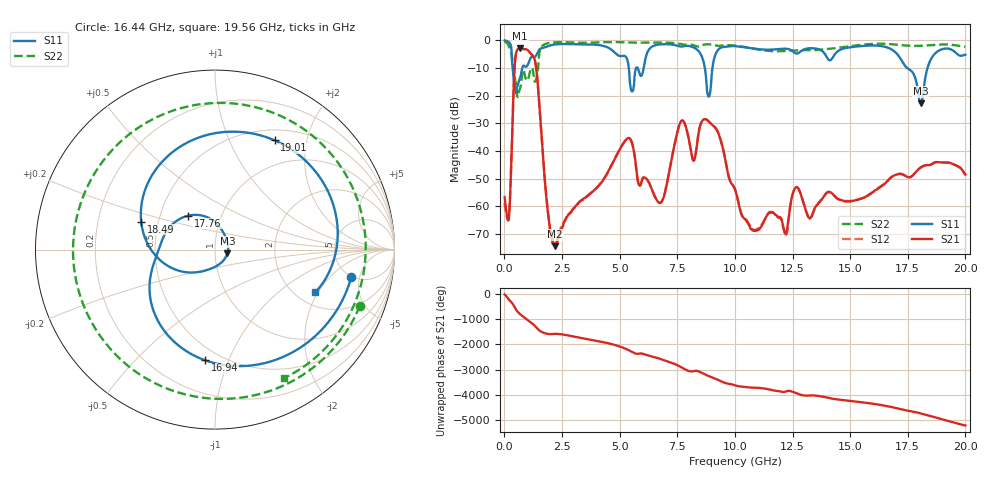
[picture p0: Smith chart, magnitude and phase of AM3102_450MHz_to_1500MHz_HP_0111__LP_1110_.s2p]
!Agilent Technologies,E8364B,MY43040894,A.07.50.67
!Agilent E8364B: A.07.50.67
!Date: Thursday, January 11, 2018 05:54:55
!Correction: S11(Full 2 Port(1,2))
!S21(Full 2 Port(1,2))
!S12(Full 2 Port(1,2))
!S22(Full 2 Port(1,2))
!S2P File: Measurements: S11, S21, S12, S22:
# Hz S  dB  R 50
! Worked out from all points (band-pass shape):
!   1601 points, 10 MHz to 20 GHz, reference 50 ohm
!   highest |S21| = -2.97 dB at 684.7 MHz (marker M1); lowest = -74.4 dB at 2.196 GHz (marker M2)
!   |S21| within 3 dB of the highest: 483.1 MHz to 1.265 GHz (781.5 MHz wide, 89.4 % of centre)
!   lowest |S11| = -22.9 dB at 18.06 GHz (marker M3), VSWR 1.16, Z = 57.3 - j2.44 ohm
!   |S11| at or under -10 dB: 358.2 MHz to 777.4 MHz (419.2 MHz wide, 73.8 % of centre); 8.697 GHz to 9.025 GHz (328.6 MHz wide, 3.71 % of centre); 17.47 GHz to 18.36 GHz (889.4 MHz wide, 4.97 % of centre)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
!   |S22| runs from -20.5 to -0.5 dB; largest |S21 - S12| = 0.0015
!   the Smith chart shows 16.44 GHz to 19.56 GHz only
!   S11 on the Smith chart (normalised r, x): 16.44 GHz: 4.90, -3.77; 16.94 GHz: 0.41, -0.83; 17.76 GHz: 0.70, +0.28; 18.49 GHz: 0.40, +0.16; 19.01 GHz: 0.64, +1.49; 19.56 GHz: 2.50, -1.89
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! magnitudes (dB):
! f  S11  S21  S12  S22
! 10 MHz  -0.1  -56.7  -58.9  -0.5
! 197.4 MHz  -0.7  -64.1  -63.4  -2.3
! 472.3 MHz  -17.8  -6.8  -6.8  -14.3
! 684.7 MHz  -13.5  -3.0  -3.0  -17.4
! 1.347 GHz  -5.8  -8.2  -8.2  -14.8
! 2.196 GHz  -1.5  -74.4  -73.7  -0.7
! 3.346 GHz  -1.5  -57.8  -57.9  -0.9
! 5.382 GHz  -9.0  -35.3  -35.3  -0.8
! 6.682 GHz  -1.6  -58.5  -58.5  -0.8
! 7.706 GHz  -2.3  -29.0  -29.0  -1.4
! 8.868 GHz  -20.3  -29.4  -29.4  -1.5
! 10.01 GHz  -2.1  -53.9  -53.9  -1.9
! 13.34 GHz  -2.9  -63.4  -63.5  -3.6
! 16.44 GHz  -2.2  -52.3  -52.2  -1.3
! 16.68 GHz  -2.8  -50.4  -50.3  -1.3
! 16.94 GHz  -4.2  -48.8  -48.8  -1.5
! 17.76 GHz  -12.4  -48.5  -48.5  -2.0
! 18.06 GHz  -22.9  -45.9  -46.0  -2.0
! 18.49 GHz  -7.1  -45.0  -45.0  -1.8
! 19.01 GHz  -3.2  -44.2  -44.3  -1.5
! 19.56 GHz  -4.3  -45.2  -45.1  -1.8
! 20 GHz  -5.2  -48.5  -48.6  -2.3
